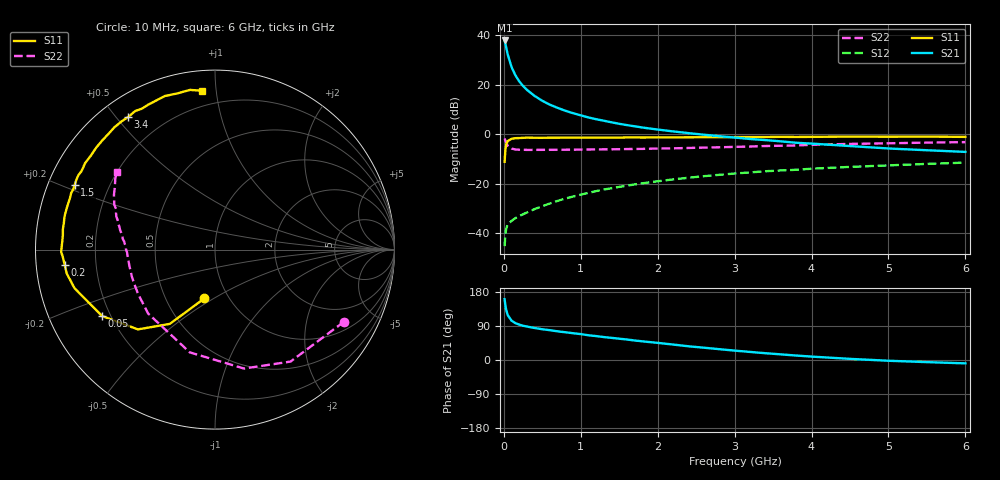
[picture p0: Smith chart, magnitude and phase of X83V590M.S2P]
! SIEMENS Small Signal Semiconductors
! BFP136W
! Si NPN RF Bipolar Junction Transistor in SOT343
! VCE = 3.5 V  IC = 90 mA
! Common Emitter S-Parameters:  September  1994
# GHz  S  MA  R  50
!  f  S11  S21  S12  S22
! GHz  MAG  ANG  MAG  ANG  MAG  ANG  MAG  ANG
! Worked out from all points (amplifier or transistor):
!   40 points, 10 MHz to 6 GHz, reference 50 ohm
!   highest |S21| = 37.9 dB at 10 MHz (marker M1)
!   |S21| within 3 dB of that: start of sweep to 31.97 MHz
!   unconditionally stable (mu >= 1): 527.1 MHz to 2.903 GHz
!   at 200 MHz: K = 0.67, MSG = 27.2 dB, |S12| = -33.0 dB
!   at 1.5 GHz: K = 1.10, MAG = 10.8 dB, |S12| = -21.2 dB
!   at 6 GHz: K = 0.96, MSG = 2.2 dB, |S12| = -11.4 dB
!   S11 on the Smith chart (normalised r, x): 10 MHz: 0.77, -0.45; 50 MHz: 0.17, -0.27; 200 MHz: 0.09, -0.05; 1.5 GHz: 0.08, +0.22; 3.4 GHz: 0.08, +0.54; 6 GHz: 0.11, +0.92
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0.01  0.2785 -102.3  78.89 160.6  0.0055 69.7  0.8236 -29.2
0.02  0.4843 -121.3  68.04 144.4  0.0095 57.9  0.7525 -56.0
0.03  0.618 -134.0  57.72 132.7  0.0123 48.4  0.6821 -76.3
0.05  0.7298 -149.5  41.35 118.5  0.0152 38.8  0.5896 -103.8
0.1  0.8115 -164.6  22.94 103.8  0.0178 35.5  0.5154 -136.2
0.15  0.837 -170.9  15.62 97.3  0.0203 38.4  0.4947 -149.8
0.2  0.8418 -174.3  11.76 93.4  0.0223 40.7  0.4888 -157.3
0.25  0.8494 -177.4  9.476 90.4  0.0243 43.7  0.487 -162.0
0.3  0.8573 -179.1  7.923 88.3  0.0264 46.6  0.4853 -165.2
0.4  0.8523 177.1  5.971 84.4  0.0309 50.9  0.4854 -169.4
0.5  0.8514 174.5  4.758 81.2  0.0353 53.8  0.486 -172.3
0.6  0.8551 172.4  3.969 78.6  0.0402 56.1  0.4867 -174.1
0.7  0.855 169.9  3.423 75.6  0.0453 58.4  0.4878 -175.5
0.9  0.8583 166.4  2.676 70.6  0.0554 59.6  0.4899 -178.1
1.1  0.8574 162.0  2.192 65.2  0.0657 60.4  0.4939 -179.7
1.5  0.8604 155.4  1.633 56.2  0.0868 59.9  0.5007 177.1
2.2  0.8674 143.0  1.146 40.8  0.1228 55.1  0.5216 171.8
3.2  0.8838 126.2  0.806 21.3  0.1701 45.9  0.5672 163.1
3.4  0.883 123.2  0.765 17.9  0.1796 43.8  0.5807 161.3
4.5  0.9001 108.1  0.58 3.0  0.2199 33.6  0.6406 151.5
5.5  0.9006 98.9  0.477 -5.6  0.2526 25.8  0.6811 144.7
6  0.888 94.6  0.442 -8.9  0.2687 21.4  0.6967 141.7
